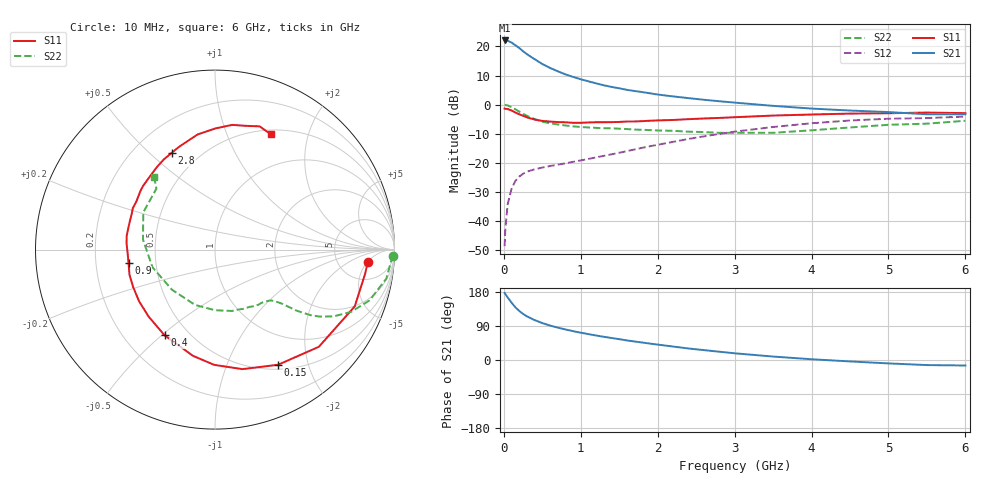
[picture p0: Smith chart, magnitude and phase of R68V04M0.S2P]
! SIEMENS Small Signal Semiconductors
! BFR193
! Si NPN RF Bipolar Junction Transistor in SOT23
! VCE = 8 V  IC = 4 mA
! Common Emitter S-Parameters:  May  1996
# GHz  S  MA  R  50
!  f  S11  S21  S12  S22
! GHz  MAG  ANG  MAG  ANG  MAG  ANG  MAG  ANG
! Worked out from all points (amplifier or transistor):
!   36 points, 10 MHz to 6 GHz, reference 50 ohm
!   highest |S21| = 22.0 dB at 10 MHz (marker M1)
!   |S21| within 3 dB of that: start of sweep to 218.4 MHz
!   unconditionally stable (mu >= 1): 976.5 MHz to 2.03 GHz
!   at 250 MHz: K = 0.36, MSG = 21.0 dB, |S12| = -23.8 dB
!   at 1.4 GHz: K = 1.07, MAG = 9.9 dB, |S12| = -17.1 dB
!   at 6 GHz: K = 0.97, MSG = 0.4 dB, |S12| = -4.1 dB
!   S11 on the Smith chart (normalised r, x): 10 MHz: 10, -5; 150 MHz: 0.56, -1.54; 400 MHz: 0.37, -0.51; 900 MHz: 0.35, -0.07; 2.8 GHz: 0.36, +0.59; 6 GHz: 0.55, +1.45
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0.01  0.8536 -4.6  12.66 177.1  0.0037 86.7  0.9921 -1.9
0.02  0.8478 -8.9  12.47 173.8  0.0075 84.8  0.9831 -3.8
0.05  0.8404 -22.1  12.51 165.0  0.0195 78.9  0.9684 -9.6
0.1  0.7925 -43.1  11.66 151.4  0.0356 69.2  0.9065 -18.2
0.15  0.7316 -61.3  10.46 139.0  0.0489 60.8  0.8336 -24.6
0.2  0.6832 -77.1  9.395 129.5  0.058 55.0  0.7582 -29.4
0.25  0.6422 -90.4  8.259 121.6  0.0649 50.8  0.6928 -32.6
0.3  0.6042 -101.8  7.353 115.2  0.0704 48.3  0.6446 -34.5
0.4  0.5539 -120.5  6.032 105.4  0.0774 45.0  0.5649 -36.9
0.5  0.5255 -134.7  4.989 97.4  0.0829 44.5  0.5096 -38.1
0.6  0.5117 -145.8  4.269 91.0  0.088 45.0  0.4784 -39.0
0.7  0.5015 -155.4  3.743 85.5  0.093 46.0  0.457 -39.9
0.9  0.4876 -171.1  2.995 76.1  0.1039 49.3  0.4228 -42.1
1.1  0.4937 176.2  2.511 68.2  0.1166 52.8  0.4053 -45.5
1.3  0.4977 166.0  2.15 61.2  0.1318 55.5  0.3931 -49.2
1.6  0.5129 153.2  1.791 51.6  0.1587 58.5  0.3803 -56.3
2.2  0.5452 131.9  1.383 35.5  0.2292 59.1  0.3548 -74.5
2.8  0.5906 114.1  1.143 21.9  0.3139 53.7  0.3275 -99.6
3.5  0.6488 98.6  0.952 9.1  0.4126 43.3  0.3279 -137.2
4.5  0.7014 82.1  0.791 -3.8  0.5336 25.8  0.405 172.1
5.5  0.7303 70.1  0.683 -13.4  0.587 7.9  0.471 133.9
6  0.7142 64.3  0.683 -14.5  0.6241 2.8  0.5277 130.0
